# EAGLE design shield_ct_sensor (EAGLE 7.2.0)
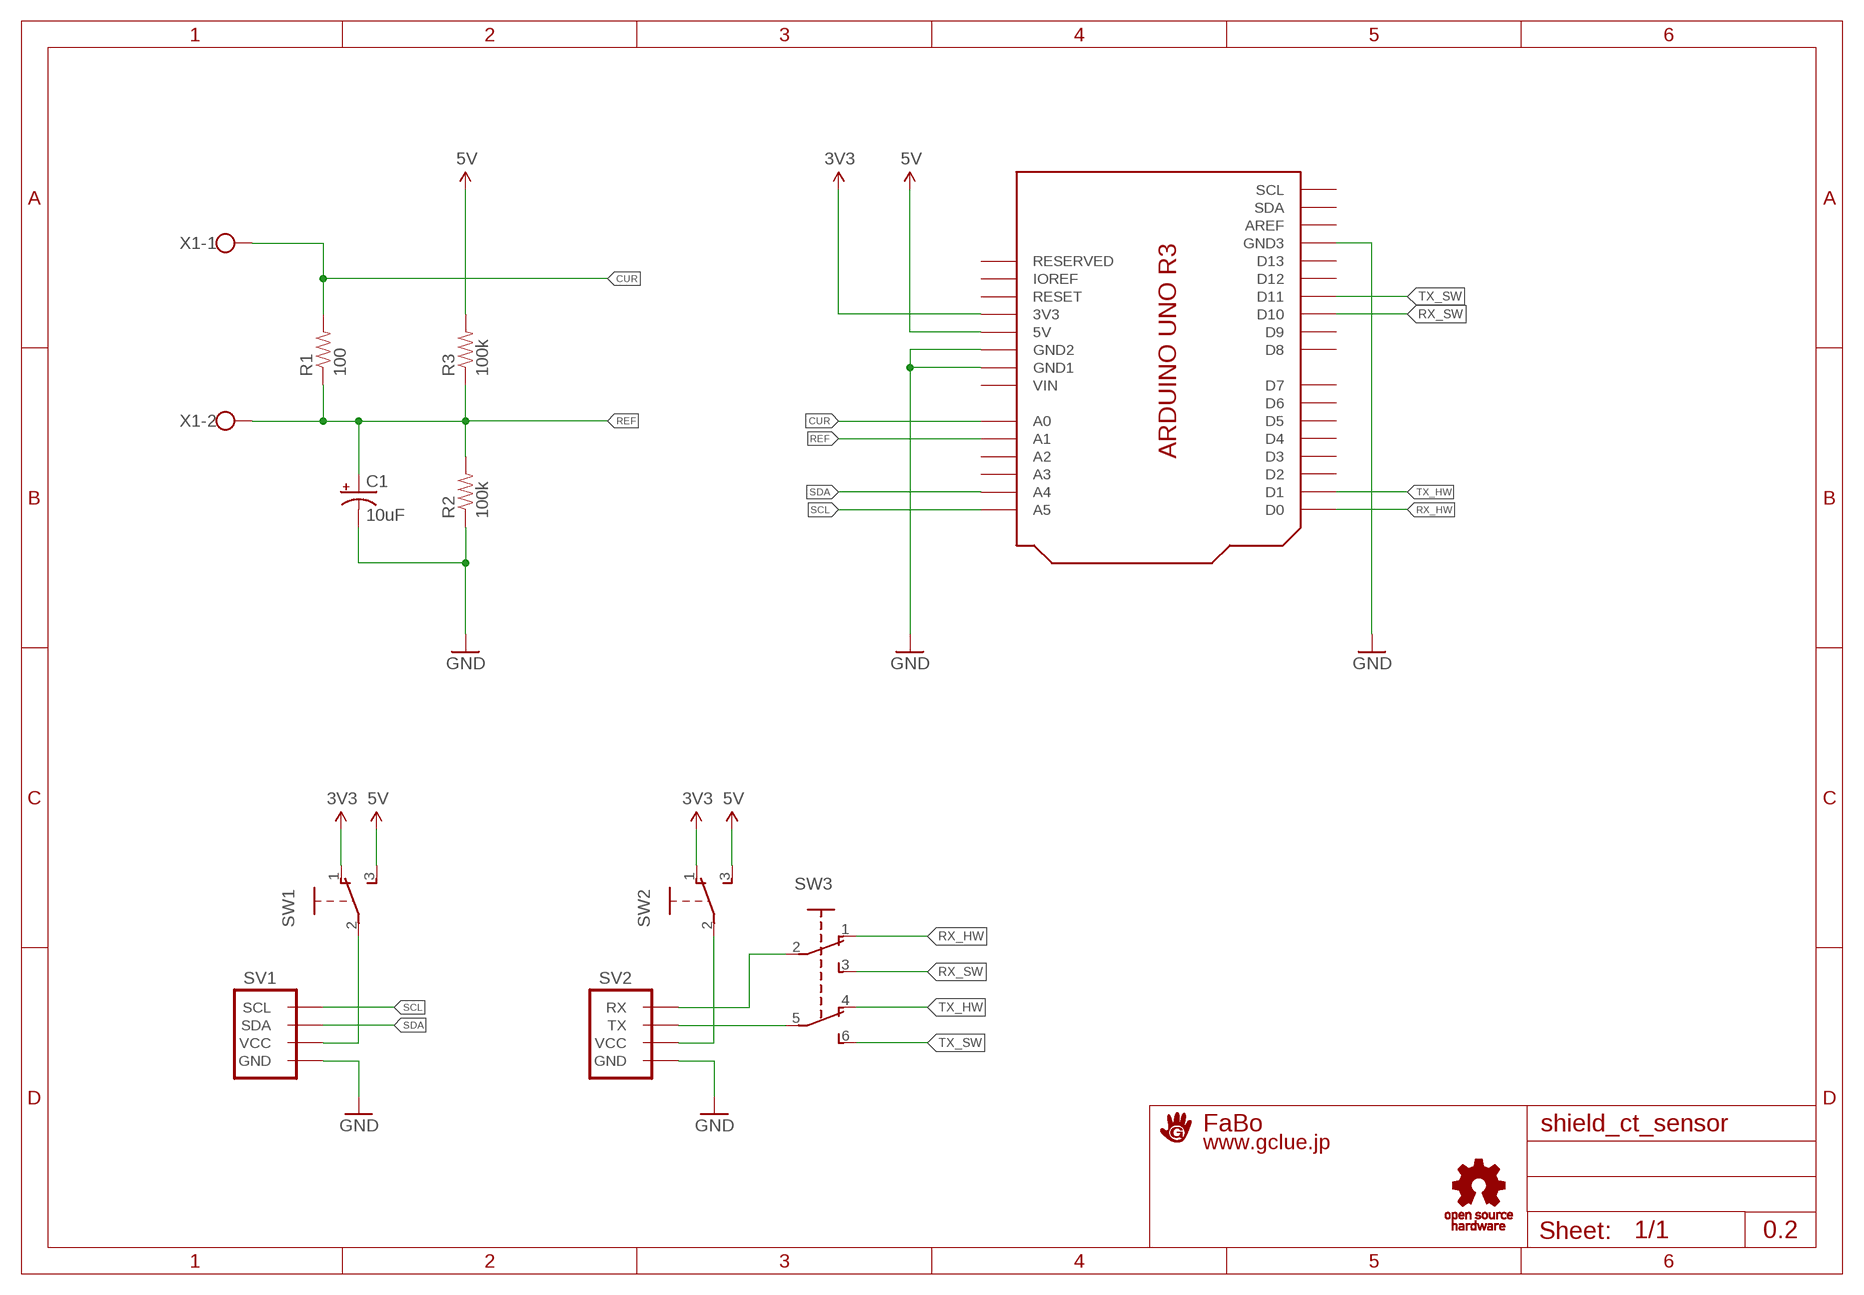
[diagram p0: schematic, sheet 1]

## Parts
C1  10uF  CAP_POL-AXL-5MM  [CAP-POL-AXL-5MM]
R1  100  RES-PTH-REGULAR  [RES-AXL-REGULAR]
R2  100k  RES-PTH-REGULAR  [RES-AXL-REGULAR]
R3  100k  RES-PTH-REGULAR  [RES-AXL-REGULAR]
SV1  BRICK_I2C_CONNECTOR  [BRICK_I2C_CONNECTOR]
SV2  BRICK_SERIAL_CONNECTOR  [BRICK_SERIAL_CONNECTOR]
SW1  SWITCH-SLIDE-EG1218  [EG1218]
SW2  SWITCH-SLIDE-EG1218  [EG1218]
SW3  SWITCH-SLIDE_2C2P-SS22F06G5-G  [SS22F06G5-G]
U1  ARDUINO_UNO_R3_SHIELD  [ARDUINO_UNO_R3]
U$2  LOGO_GCLUE-M  [LOGO_GCLUE_M]
U$3  LOGO_OSHW_T-M  [LOGO_OSHW_T_M]
X1  W237-102  [W237-102]

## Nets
3V3: SW1.1 SW2.1 U1.3V3
5V: R3.P$2 SW1.3 SW2.3 U1.5V
CUR: R1.P$2 U1.A0 X1.1
GND: C1.- R2.P$1 SV1.GND SV2.GND U1.GND1 U1.GND2 U1.GND3
N$1: SV2.VCC SW2.2
N$2: SV1.VCC SW1.2
N$3: SV2.TX SW3.5
N$4: SV2.RX SW3.2
REF: C1.+ R1.P$1 R2.P$2 R3.P$1 U1.A1 X1.2
RX_HW: SW3.1 U1.D0
RX_SW: SW3.3 U1.D10
SCL: SV1.SCL U1.A5
SDA: SV1.SDA U1.A4
TX_HW: SW3.4 U1.D1
TX_SW: SW3.6 U1.D11
Unconnected: U1.A2 U1.A3 U1.AREF U1.D2 U1.D3 U1.D4 U1.D5 U1.D6 U1.D7 U1.D8 U1.D9 U1.D12 U1.D13 U1.IOREF U1.RESERVED U1.RESET U1.SCL U1.SDA

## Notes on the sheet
- 0.2

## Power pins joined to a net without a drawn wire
VIN: U1.VIN

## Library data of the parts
C1 = GClue:CAP_POL: Capacitor Polarized
R1-R3 = GClue:RES
SV1 = GClue:BRICK_I2C_CONNECTOR: Brick Connector female for OUT/IN Shield
SV2 = GClue:BRICK_SERIAL_CONNECTOR
SW1 SW2 = GClue:SWITCH-SLIDE
SW3 = GClue:SWITCH-SLIDE_2C2P
U1 = GClue:ARDUINO_UNO_R3_SHIELD
U$2 = GClue:LOGO_GCLUE
U$3 = GClue:LOGO_OSHW_T
X1 = con-wago-500:W237-102: WAGO SCREW CLAMP; MPN: 237-102; OC_FARNELL: unknown; OC_NEWARK: 70K9898

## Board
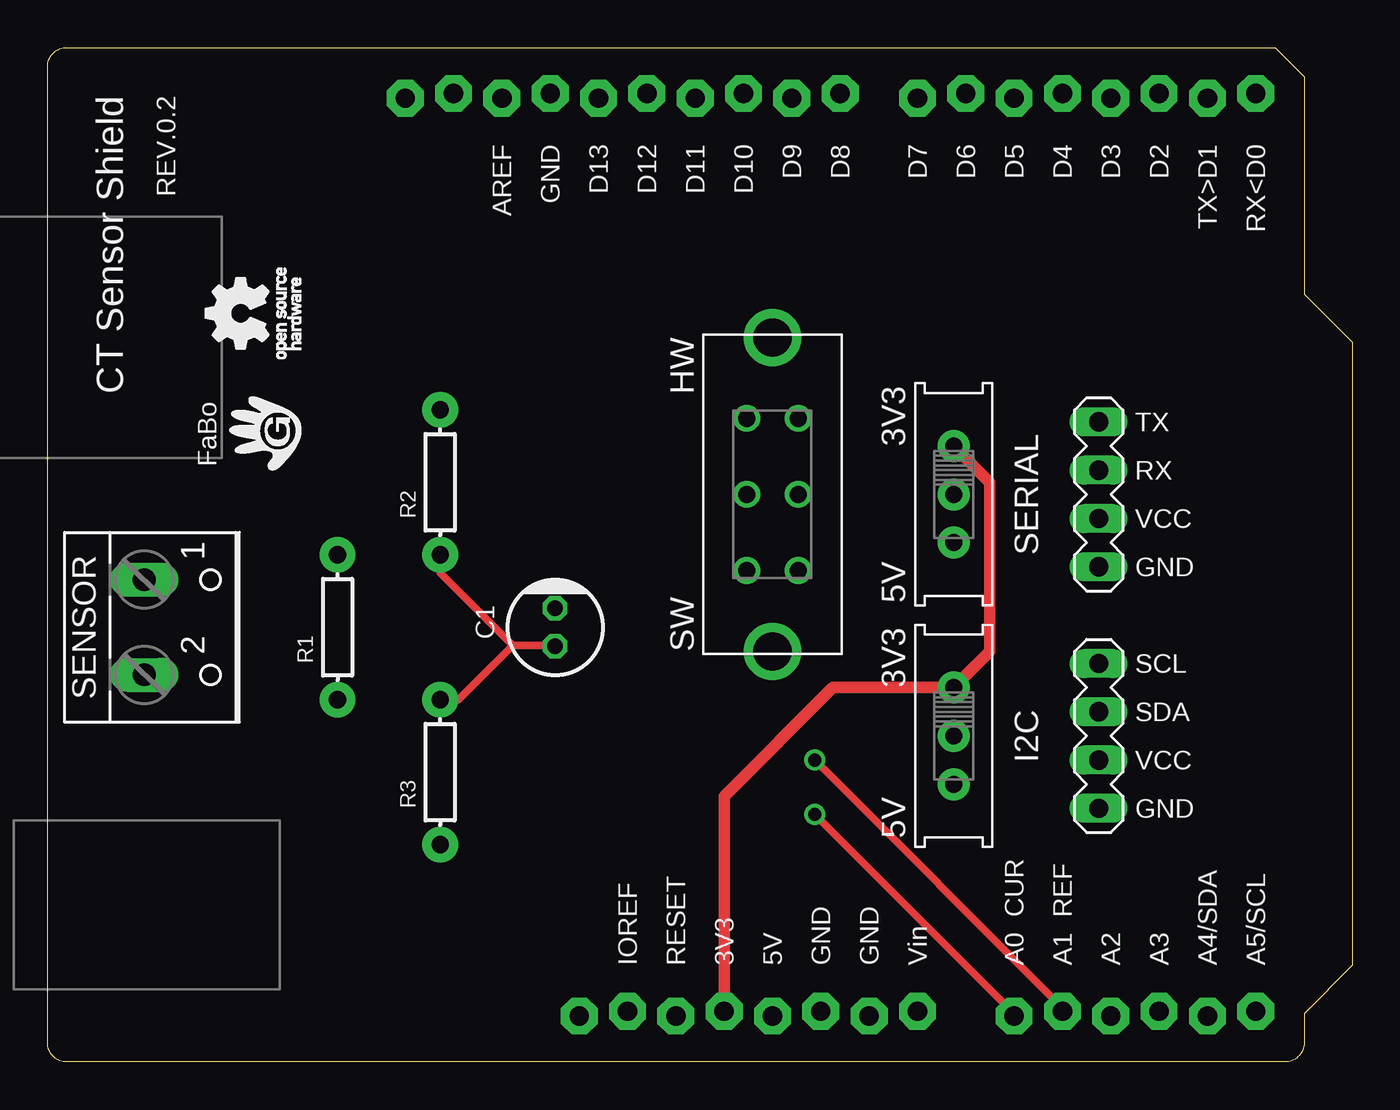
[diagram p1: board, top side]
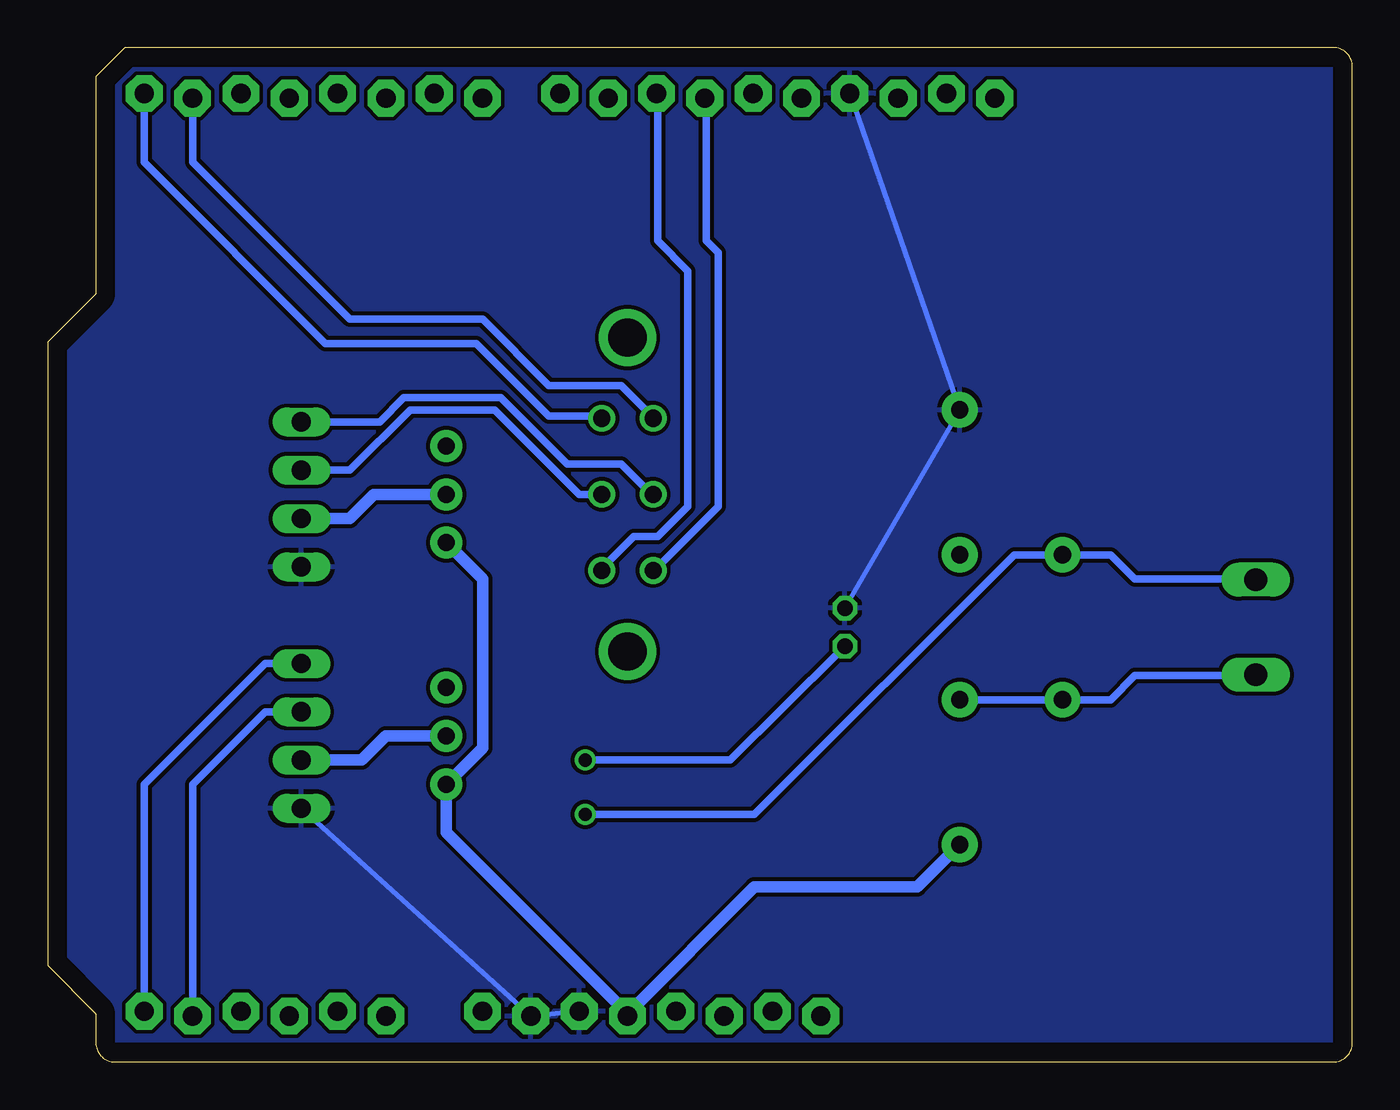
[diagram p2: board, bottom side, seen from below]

Size 68.58 x 53.34 mm. Coordinates in mm from the lower left corner, seen from the top.
Copper layers (1*16): Top 0.035mm / dielectric 1.5mm / Bottom 0.035mm
Design rules "default": minimum track width 10mil, minimum drill 24mil, track to track 8mil, track to pad 8mil, pad to pad 8mil, via to via 8mil, smd to smd 8mil, copper to edge 40mil, drill to drill 8mil, minimum pad ring 10mil, minimum via ring 8mil, stop-mask expansion 4mil, vias tented up to drill 0mil, thermal gap 10mil

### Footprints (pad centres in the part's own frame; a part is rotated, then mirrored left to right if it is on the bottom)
CAP-POL-AXL-5MM = drill 0.8 octagon: + 1,0; - -1,0
RES-AXL-REGULAR = drill 0.9 pad 1.88: P$1 -3.81,0; P$2 3.81,0
BRICK_I2C_CONNECTOR = drill 1.016 long: GND -3.81,0; SCL 3.81,0; SDA 1.27,0; VCC -1.27,0
BRICK_SERIAL_CONNECTOR = drill 1.016 long: GND -3.81,0; RX 1.27,0; TX 3.81,0; VCC -1.27,0
EG1218 = drill 0.9 pad 1.676: 1 -2.54,0; 2 0,0; 3 2.54,0
SS22F06G5-G = drill 0.9: 1 -4,1.35; 2 0,1.35; 3 4,1.35; 4 -4,-1.35; 5 0,-1.35; 6 4,-1.35 | drill 2: P$1 8.25,0; P$5 -8.25,0
ARDUINO_UNO_R3 = drill 1.016 pad 1.93 octagon: 3V3 35.56,2.667; 5V 38.1,2.413; A0 50.8,2.413; A1 53.34,2.667; A2 55.88,2.413; A3 58.42,2.667; A4 60.96,2.413; A5 63.5,2.667; AREF 23.876,50.673; D0 63.5,50.927; D1 60.96,50.673; D2 58.42,50.927; D3 55.88,50.673; D4 53.34,50.927; D5 50.8,50.673; D6 48.26,50.927; D7 45.72,50.673; D8 41.656,50.927; D9 39.116,50.673; D10 36.576,50.927; D11 34.036,50.673; D12 31.496,50.927; D13 28.956,50.673; GND1 43.18,2.413; GND2 40.64,2.667; GND3 26.416,50.927; IOREF 30.48,2.667; RESERVED 27.94,2.413; RESET 33.02,2.413; SCL 18.796,50.673; SDA 21.336,50.927; VIN 45.72,2.667
W237-102 = drill 1.194 long: 1 -2.5,-1.27; 2 2.5,-1.27

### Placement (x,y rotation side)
C1  26.67,22.86 270 top
R1  15.24,22.86 90 top
R2  20.64,30.48 270 top
R3  20.64,15.24 270 top
SV1  55.24,17.14 90 top
SV2  55.24,29.84 90 top
SW1  47.62,17.14 270 top
SW2  47.62,29.84 270 top
SW3  38.1,29.84 270 top
U1  0,0 0 top
U$2  11.43,33.02 90 top
U$3  10.16,39.37 90 top
X1  6.35,22.86 270 top

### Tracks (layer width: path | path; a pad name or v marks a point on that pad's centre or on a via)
3V3
  Top 0.61: U1.3V3 35.56,13.97 41.27,19.68 SW1.1 49.53,21.59 49.53,30.48 SW2.1
5V
  Bottom 0.406: U1.5V 38.1,2.54
  Bottom 0.61: R3.P$2 22.86,9.21 31.43,9.21 38.1,2.54 47.62,12.06 SW1.3 45.72,16.51 45.72,25.4 SW2.3
CUR  (via drill 0.7)
  Top 0.406: U1.A0 50.8,2.54 v40.32,13.02
  Bottom 0.406: X1.1 5.08,25.4 11.43,25.4 12.7,26.67 R1.P$2 17.78,26.67 31.43,13.02 v40.32,13.02
GND
  Bottom 0.254: U1.GND3 R2.P$1 C1.- | U1.GND2 U1.GND1 SV1.GND
  pour Bottom: -0.64,53.98 69.22,53.98 69.22,-0.64 -0.64,-0.64
N$1
  Bottom 0.61: SW2.2 51.44,29.84 52.7,28.57 SV2.VCC
N$2
  Bottom 0.61: SW1.2 50.8,17.14 52.07,15.88 SV1.VCC
N$3
  Bottom 0.406: SV2.TX 51.12,33.66 49.85,34.92 44.77,34.92 41.27,31.43 38.42,31.43 36.83,29.84 SW3.5
N$4
  Bottom 0.406: SV2.RX 52.7,31.11 49.53,34.29 45.09,34.29 40.64,29.84 SW3.2
REF  (via drill 0.7)
  Top 0.406: U1.A1 53.34,2.86 v40.32,15.88 | C1.+ 26.67,21.91 24.45,21.91 | 24.45,21.91 20.64,25.72 R2.P$2 | R3.P$1 21.59,19.05 24.45,21.91
  Bottom 0.406: X1.2 5.08,20.32 11.43,20.32 12.7,19.05 R1.P$1 R3.P$1 | C1.+ 26.99,21.54 32.7,15.88 v40.32,15.88
RX_HW
  Bottom 0.406: SW3.1 39.69,33.97 42.23,33.97 46.04,37.78 53.98,37.78 63.5,47.31 U1.D0
RX_SW
  Bottom 0.406: SW3.3 39.37,26.04 37.78,27.62 36.51,27.62 34.92,29.21 34.92,41.59 36.51,43.18 36.51,50.93 U1.D10
SCL
  Bottom 0.406: U1.A5 63.5,14.61 57.15,20.95 SV1.SCL
SDA
  Bottom 0.406: SV1.SDA 57.15,18.41 60.96,14.61 U1.A4
TX_HW
  Bottom 0.406: SW3.4 36.83,33.97 38.42,35.56 42.23,35.56 45.72,39.05 52.7,39.05 60.96,47.31 U1.D1
TX_SW
  Bottom 0.406: SW3.6 36.51,26.04 33.34,29.21 33.34,42.55 33.97,43.18 33.97,50.48 U1.D11

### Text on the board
tPlace: CT Sensor Shield | REV.0.2 | HW | 3V3 | TX | FaBo | RX | SERIAL | VCC | GND | 5V | SENSOR | 3V3 | SW | SCL | SDA | I2C | VCC | GND | 5V | CUR | REF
